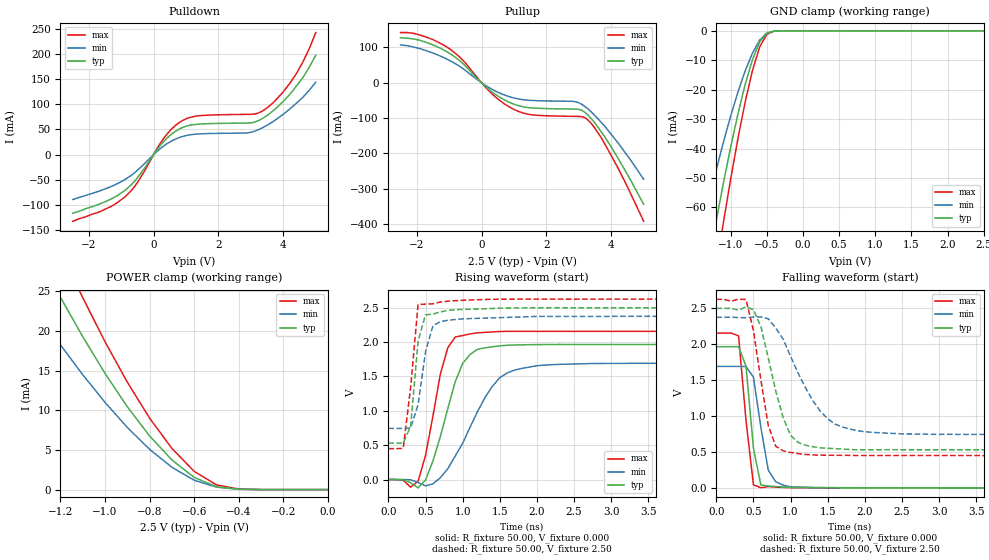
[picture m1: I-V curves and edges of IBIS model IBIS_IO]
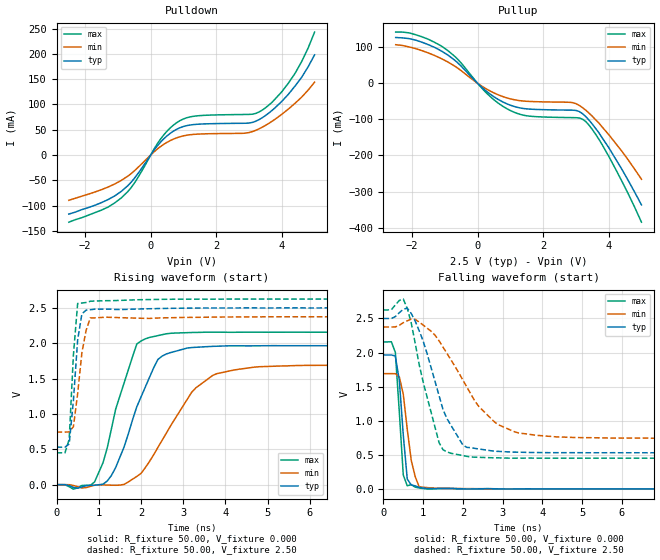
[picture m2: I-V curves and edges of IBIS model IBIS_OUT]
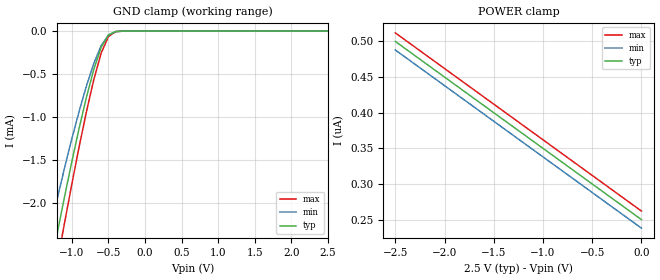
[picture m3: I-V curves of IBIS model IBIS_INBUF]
| IBIS file .ibs created by s2ibis2 version 1.1
| North Carolina State University Electronics Research Laboratory  1995
[IBIS ver]   2.1
[File name]   75602_pf.ibs
[File Rev]   1.3
[Date]   Thursday, June 28, 2001
[Source]   Integrated Device Technology, Inc.
[Notes]   1. Temperatures: typ=25C, min=100C, max=0C 2. Cemos11.5_2.5v
   process. 3. Ramp rates based on 50 ohm load.
[Copyright]   Copyright 2000, Integrated Device Technology, Inc. Integrated
   Device Technology, Inc. ("IDT") hereby grants the user of this
   IBIS model a non-exclusive, nontransferable license to use
   this IBIS model under the following terms. The user is granted
   this license only to use the IBIS model and is not granted
   rights to sell, copy (except as needed to run the IBIS model),
   rent, lease or sub-license the IBIS model in whole or in part,
   or in modified form to anyone. The User may modify the IBIS
   model to suit its specific applications, but rights to
   derivative works and such modifications shall belong to IDT.
   This IBIS model is provided on an AS IS" basis and IDT makes
   absolutely no warranty with respect to the information
   contained herein. IDT DISCLAIMS AND CUSTOMER WAIVES ALL
   WARRANTIES, EXPRESS AND IMPLIED, INCLUDING WARRANTIES OF
   MERCHANTABILITY AND FITNESS FOR A PARTICULAR PURPOSE. THE
   ENTIRE RISK AS TO QUALITY AND PERFORMANCE IS WITH THE USER
   ACCORDINGLY, IN NO EVENT SHALL IDT BE LIABLE FOR ANY DIRECT OR
   INDIRECT DAMAGES, WHETHER IN CONTRACT OR TORT, INCLUDING ANY
   LOST PROFITS OR OTHER INCIDENTAL, CONSEQUENTIAL, EXEMPLARY, OR
   PUNITIVE DAMAGES ARISING OUT OF THE USE OR APPLICATION OF THE
   IBIS model. Further, IDT reserves the right to make changes
   without notice to any product herein to improve reliability,
   function, or design. IDT does not convey any license under
   patent rights or any other intellectual property rights,
   including those of third parties. IDT is not obligated to
   provide maintenance or support for the licensed IBIS model.
|   Component IDT71T75602z_PIPELINE_ZBT_SRAM
[Component]   IDT71T75602z
[Manufacturer]   Integrated Device Technology
|   IBIS model for (PF) 100-TQFP package
[Package]
| variable   typ   min   max
R_pkg   10.00m   9.00m   11.00m
L_pkg   5.50nH   5.00nH   5.60nH
C_pkg   0.40pF   0.30pF   0.47pF
[Pin]  signal_name   model_name   R_pin   L_pin   C_pin
1   I/OP3   IBIS_IO
2   I/O16   IBIS_IO
3   I/O17   IBIS_IO
4   VDDQ   POWER
5   VSS   GND
6   I/O18   IBIS_IO
7   I/O19   IBIS_IO
8   I/O20   IBIS_IO
9   I/O21   IBIS_IO
10   VSS   GND
11   VDDQ   POWER
12   I/O22   IBIS_IO
13   I/O23   IBIS_IO
14   VDD   POWER
15   VDD   POWER
16   VDD   POWER
17   VSS   GND
18   I/O24   IBIS_IO
19   I/O25   IBIS_IO
20   VDDQ   POWER
21   VSS   GND
22   I/O26   IBIS_IO
23   I/O27   IBIS_IO
24   I/O28   IBIS_IO
25   I/O29   IBIS_IO
26   VSS   GND
27   VDDQ   POWER
28   I/O30   IBIS_IO
29   I/O31   IBIS_IO
30   I/OP4   IBIS_IO
31   LBO/   IBIS_INBUF
32   A5   IBIS_INBUF
33   A4   IBIS_INBUF
34   A3   IBIS_INBUF
35   A2   IBIS_INBUF
36   A1   IBIS_INBUF
37   A0   IBIS_INBUF
38   TMS   IBIS_INBUF
39   TDI   IBIS_INBUF
40   VSS   GND
41   VDD   POWER
42   TDO   IBIS_OUT
43   TCK   IBIS_INBUF
44   A10   IBIS_INBUF
45   A11   IBIS_INBUF
46   A12   IBIS_INBUF
47   A13   IBIS_INBUF
48   A14   IBIS_INBUF
49   A15   IBIS_INBUF
50   A16   IBIS_INBUF
51   I/OP1   IBIS_IO
52   I/O0   IBIS_IO
53   I/O1   IBIS_IO
54   VDDQ   POWER
55   VSS   GND
56   I/O2   IBIS_IO
57   I/O3   IBIS_IO
58   I/O4   IBIS_IO
59   I/O5   IBIS_IO
60   VSS   GND
61   VDDQ   POWER
62   I/O6   IBIS_IO
63   I/O7   IBIS_IO
64   ZZ   IBIS_INBUF
65   VDD   POWER
66   VDD   POWER
67   VSS   GND
68   I/O8   IBIS_IO
69   I/O9   IBIS_IO
70   VDDQ   POWER
71   VSS   GND
72   I/O10   IBIS_IO
73   I/O11   IBIS_IO
74   I/O12   IBIS_IO
75   I/O13   IBIS_IO
76   VSS   GND
77   VDDQ   POWER
78   I/O14   IBIS_IO
79   I/O15   IBIS_IO
80   I/OP2   IBIS_IO
81   A9   IBIS_INBUF
82   A8   IBIS_INBUF
83   A17   IBIS_INBUF
84   A18   IBIS_INBUF
85   ADV/LD/   IBIS_INBUF
86   OE/   IBIS_INBUF
87   CEN/   IBIS_INBUF
88   R/W/   IBIS_INBUF
89   CLK   IBIS_INBUF
90   VSS   GND
91   VDD   POWER
92   CE2/   IBIS_INBUF
93   BW1/   IBIS_INBUF
94   BW2/   IBIS_INBUF
95   BW3/   IBIS_INBUF
96   BW4/   IBIS_INBUF
97   CE2   IBIS_INBUF
98   CE1/   IBIS_INBUF
99   A7   IBIS_INBUF
100   A6   IBIS_INBUF
| Models and submodels in the file (3): IBIS_IO (I/O), IBIS_OUT (Output), IBIS_INBUF (Input)
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| in   in   dummy_model
| oel  oel   dummy_model
| int  int   dummy_model
| oelt oelt   dummy_model
|   Model IBIS_IO
[Model]   IBIS_IO
Model_type   I/O
Polarity   Non-Inverting
Enable   Active-Low
Vinl =  0.700V
Vinh =  1.700V
Vmeas =  1.250V
Cref =  0.000F
Rref = 50.000
Vref =  1.250V
C_comp   3.00pF   2.00pF   4.00pF
[Temperature Range]   25.00   100.00   0.000
[Voltage Range]   2.50V   2.37V   2.62V
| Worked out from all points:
|   slope of the pulldown table from 0 to 0.375 V, typ, clamps not added: 12.4 ohm
|   slope of the pullup table from 0 to 0.375 V, typ, clamps not added: 12.8 ohm
|   GND clamp passes 1 mA (typ) near -0.51 V on its own axis
|   POWER clamp passes 1 mA (typ) near -0.55 V on its own axis
|   rising waveform, R_fixture 50.00, V_fixture 0.000: 20-80 % time 321ps typ, 500ps min, 235ps max; typ from 0 V to 1.97 V
|   rising waveform, R_fixture 50.00, V_fixture 2.50: 20-80 % time 112ps typ, 156ps min, 122ps max; typ from 0.53 V to 2.5 V
|   falling waveform, R_fixture 50.00, V_fixture 0.000: 20-80 % time 121ps typ, 158ps min, 123ps max; typ from 1.97 V to 0 V
|   falling waveform, R_fixture 50.00, V_fixture 2.50: 20-80 % time 289ps typ, 489ps min, 197ps max; typ from 2.5 V to 0.53 V
[Pulldown]
| voltage   I(typ)   I(min)   I(max)
-2.5V     -117mA     -89.7mA    -133mA
-1.7V     -99.4mA    -73.2mA    -115mA
-900mV    -72.13mA   -50.4mA    -85.16mA
-500mV    -46.26mA   -31.43mA   -55.78mA
300mV     25.33mA    16.62mA    31.45mA
900mV     54.03mA    36.14mA    68.11mA
1.5V      61mA       41.41mA    77.8mA
3V        63.11mA    44.29mA    80.16mA
3.5V      77.88mA    58.43mA    93.16mA
4V        106mA      80.39mA    125mA
4.4V      136mA      102mA      161mA
5V        198mA      144mA      243mA
[Pullup]
| voltage   I(typ)   I(min)   I(max)
-2.5V     127mA      107mA      142mA
-1.9V     120mA      96.48mA    135mA
-1.1V     89.31mA    68.24mA    103mA
-600mV    56.27mA    41.71mA    66.02mA
300mV     -24.21mA   -17.31mA   -29.47mA
1V        -60.72mA   -43.11mA   -75.48mA
1.6V      -71.56mA   -50.32mA   -91.16mA
2.9V      -74.5mA    -53.66mA   -95.14mA
3.2V      -84.55mA   -67.99mA   -99.54mA
3.5V      -114mA     -92.99mA   -129mA
3.8V      -153mA     -123mA     -173mA
5V        -344mA     -273mA     -392mA
[GND_clamp]
| voltage   I(typ)   I(min)   I(max)
-2.5V     -256mA     -196mA     -298mA
-1.4V     -91.8mA    -67.57mA   -112mA
-1.3V     -77.92mA   -57.18mA   -96.09mA
-1.2V     -64.46mA   -47.2mA    -80.22mA
-1.1V     -51.57mA   -37.73mA   -64.88mA
-900mV    -28.17mA   -20.77mA   -36.54mA
-800mV    -18.18mA   -13.58mA   -24.15mA
-700mV    -9.823mA   -7.577mA   -13.54mA
-600mV    -3.759mA   -3.157mA   -5.506mA
-500mV    -740uA     -782uA     -1.15mA
-300mV    -2.842uA   -8.572uA   -3.594uA
2.5V      250nA      281nA      250nA
[POWER_clamp]
| voltage   I(typ)   I(min)   I(max)
-2.5V     100mA      78.58mA    117mA
-1.4V     34.98mA    26.45mA    42.72mA
-1.3V     29.51mA    22.26mA    36.31mA
-1.2V     24.26mA    18.26mA    30.12mA
-1.1V     19.29mA    14.49mA    24.21mA
-900mV    10.45mA    7.838mA    13.55mA
-800mV    6.77mA     5.078mA    9.014mA
-700mV    3.737mA    2.813mA    5.196mA
-600mV    1.535mA    1.182mA    2.3mA
-500mV    362uA      310uA      599uA
-400mV    41.18uA    46.02uA    69.44uA
0V        250nA      239nA      262nA
[Ramp]
| variable   typ   min   max
dV/dt_r   1.18/0.30n   1.02/0.49n   1.30/0.22n
dV/dt_f   1.18/0.28n   0.98/0.50n   1.31/0.21n
R_load = 50.00
[Rising Waveform]
R_fixture = 50.00
V_fixture = 0.000
V_fixture_min = 0.000
V_fixture_max = 0.000
C_fixture = 0.000F
R_dut = 68.00m
L_dut = 2.31nH
C_dut = 0.65pF
| time   V(typ)   V(min)   V(max)
0s        0V         0V         0V
300ps     -45.68mV   -3.202mV   -111mV
400ps     -121mV     -43.62mV   -25.43mV
500ps     -8.692mV   -91.97mV   351mV
700ps     627mV      26.44mV    1.537V
800ps     1.032V     157mV      1.917V
1.1ns     1.819V     763mV      2.119V
1.5ns     1.945V     1.482V     2.154V
2ns       1.963V     1.656V     2.156V
9.9ns     1.965V     1.691V     2.156V
[Rising Waveform]
R_fixture = 50.00
V_fixture = 2.50
V_fixture_min = 2.37
V_fixture_max = 2.62
C_fixture = 0.000F
R_dut = 68.00m
L_dut = 2.31nH
C_dut = 0.65pF
| time   V(typ)   V(min)   V(max)
0s        530mV      744mV      450mV
200ps     530mV      744mV      453mV
300ps     777mV      750mV      1.343V
400ps     2.017V     1.09V      2.547V
500ps     2.397V     1.859V     2.552V
600ps     2.407V     2.239V     2.557V
700ps     2.44V      2.298V     2.583V
800ps     2.46V      2.318V     2.595V
2ns       2.499V     2.373V     2.625V
9.9ns     2.5V       2.375V     2.625V
[Falling Waveform]
R_fixture = 50.00
V_fixture = 0.000
V_fixture_min = 0.000
V_fixture_max = 0.000
C_fixture = 0.000F
R_dut = 68.00m
L_dut = 2.31nH
C_dut = 0.65pF
| time   V(typ)   V(min)   V(max)
0s        1.965V     1.691V     2.156V
200ps     1.965V     1.691V     2.156V
300ps     1.966V     1.691V     2.116V
400ps     1.694V     1.689V     939mV
500ps     556mV      1.541V     41.85mV
600ps     40.07mV    844mV      1.621mV
700ps     25.66mV    246mV      17.7mV
800ps     17.72mV    84.79mV    10.16mV
1ns       6.48mV     15.89mV    3.136mV
9.9ns     -347nV     1.011uV    -1.87uV
[Falling Waveform]
R_fixture = 50.00
V_fixture = 2.50
V_fixture_min = 2.37
V_fixture_max = 2.62
C_fixture = 0.000F
R_dut = 68.00m
L_dut = 2.31nH
C_dut = 0.65pF
| time   V(typ)   V(min)   V(max)
0s        2.5V       2.375V     2.625V
400ps     2.52V      2.368V     2.623V
500ps     2.481V     2.379V     2.19V
600ps     2.246V     2.381V     1.503V
700ps     1.808V     2.354V     867mV
800ps     1.349V     2.225V     580mV
1ns       730mV      1.83V      492mV
1.5ns     551mV      961mV      454mV
2ns       530mV      781mV      450mV
9.9ns     530mV      744mV      450mV
|   Model IBIS_OUT
[Model]   IBIS_OUT
Model_type   Output
Polarity   Non-Inverting
Enable   Active-Low
Vmeas =  1.250V
Cref =  0.000F
Rref = 50.000
Vref =  1.250V
C_comp   3.00pF   2.00pF   4.00pF
[Temperature Range]   25.00   100.00   0.000
[Voltage Range]   2.50V   2.37V   2.62V
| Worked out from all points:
|   slope of the pulldown table from 0 to 0.375 V, typ, clamps not added: 12.4 ohm
|   slope of the pullup table from 0 to 0.375 V, typ, clamps not added: 12.8 ohm
|   rising waveform, R_fixture 50.00, V_fixture 0.000: 20-80 % time 737ps typ, 1.06ns min, 595ps max; typ from 0 V to 1.97 V
|   rising waveform, R_fixture 50.00, V_fixture 2.50: 20-80 % time 160ps typ, 204ps min, 128ps max; typ from 0.53 V to 2.5 V
|   falling waveform, R_fixture 50.00, V_fixture 0.000: 20-80 % time 159ps typ, 227ps min, 143ps max; typ from 1.97 V to 0 V
|   falling waveform, R_fixture 50.00, V_fixture 2.50: 20-80 % time 675ps typ, 1.11ns min, 525ps max; typ from 2.5 V to 0.53 V
[Pulldown]
| voltage   I(typ)   I(min)   I(max)
-2.5V     -117mA     -89.7mA    -133mA
-1.5V     -94.2mA    -68.59mA   -109mA
-900mV    -72.12mA   -50.41mA   -85.11mA
-500mV    -46.26mA   -31.43mA   -55.77mA
300mV     25.33mA    16.62mA    31.45mA
900mV     54.03mA    36.14mA    68.11mA
1.5V      61mA       41.41mA    77.8mA
3V        63.11mA    44.29mA    80.16mA
3.5V      77.88mA    58.43mA    93.16mA
4V        106mA      80.39mA    125mA
4.4V      136mA      102mA      161mA
5V        198mA      144mA      243mA
[Pullup]
| voltage   I(typ)   I(min)   I(max)
-2.5V     127mA      107mA      142mA
-1.9V     120mA      96.48mA    135mA
-1.1V     89.31mA    68.24mA    103mA
-600mV    56.27mA    41.71mA    66.02mA
300mV     -24.21mA   -17.31mA   -29.47mA
1V        -60.72mA   -43.11mA   -75.48mA
1.6V      -71.56mA   -50.32mA   -91.16mA
2.9V      -74.49mA   -53.6mA    -95.14mA
3.3V      -92.23mA   -74.49mA   -106mA
3.6V      -125mA     -101mA     -141mA
4V        -178mA     -142mA     -202mA
5V        -337mA     -266mA     -385mA
[Ramp]
| variable   typ   min   max
dV/dt_r   1.18/0.74n   1.02/1.05n   1.30/0.61n
dV/dt_f   1.18/0.66n   0.98/1.11n   1.31/0.53n
R_load = 50.00
[Rising Waveform]
R_fixture = 50.00
V_fixture = 0.000
V_fixture_min = 0.000
V_fixture_max = 0.000
C_fixture = 0.000F
R_dut = 68.00m
L_dut = 2.31nH
C_dut = 0.65pF
| time   V(typ)   V(min)   V(max)
0s        0V         0V         0V
900ps     -8.624mV   -8.352mV   38.26mV
1.1ns     6.189mV    -4.095mV   309mV
1.4ns     242mV      -8.698mV   1.068V
1.9ns     1.101V     116mV      1.988V
2.1ns     1.378V     239mV      2.062V
2.5ns     1.818V     628mV      2.121V
3.2ns     1.939V     1.307V     2.152V
3.8ns     1.958V     1.571V     2.157V
9.9ns     1.965V     1.691V     2.156V
[Rising Waveform]
R_fixture = 50.00
V_fixture = 2.50
V_fixture_min = 2.37
V_fixture_max = 2.62
C_fixture = 0.000F
R_dut = 68.00m
L_dut = 2.31nH
C_dut = 0.65pF
| time   V(typ)   V(min)   V(max)
0s        530mV      744mV      450mV
200ps     530mV      744mV      450mV
300ps     576mV      745mV      642mV
400ps     1.192V     821mV      1.837V
500ps     2.047V     1.285V     2.562V
600ps     2.415V     1.865V     2.569V
700ps     2.468V     2.182V     2.577V
800ps     2.474V     2.359V     2.594V
2.9ns     2.495V     2.364V     2.624V
9.9ns     2.5V       2.375V     2.625V
[Falling Waveform]
R_fixture = 50.00
V_fixture = 0.000
V_fixture_min = 0.000
V_fixture_max = 0.000
C_fixture = 0.000F
R_dut = 68.00m
L_dut = 2.31nH
C_dut = 0.65pF
| time   V(typ)   V(min)   V(max)
0s        1.965V     1.691V     2.156V
200ps     1.965V     1.691V     2.159V
300ps     1.948V     1.69V      2.004V
400ps     1.593V     1.644V     1.13V
500ps     790mV      1.388V     203mV
600ps     144mV      875mV      45.08mV
700ps     58.18mV    420mV      62.05mV
800ps     44.52mV    179mV      25.37mV
900ps     21.3mV     29.52mV    12.94mV
9.9ns     26.72uV    503nV      67.94uV
[Falling Waveform]
R_fixture = 50.00
V_fixture = 2.50
V_fixture_min = 2.37
V_fixture_max = 2.62
C_fixture = 0.000F
R_dut = 68.00m
L_dut = 2.31nH
C_dut = 0.65pF
| time   V(typ)   V(min)   V(max)
0s        2.5V       2.375V     2.625V
500ps     2.634V     2.438V     2.785V
800ps     2.462V     2.487V     2.137V
1ns       2.169V     2.403V     1.568V
1.4ns     1.368V     2.173V     678mV
1.6ns     1.029V     1.986V     542mV
2.1ns     609mV      1.493V     477mV
2.8ns     552mV      979mV      456mV
3.4ns     538mV      821mV      451mV
9.9ns     530mV      743mV      450mV
|   Model IBIS_INBUF
[Model]   IBIS_INBUF
Model_type   Input
Vinl =  0.700V
Vinh =  1.700V
Vmeas =  1.250V
C_comp   1.00pF   0.80pF   1.20pF
[Temperature Range]   25.00   100.00   0.000
[Voltage Range]   2.50V   2.37V   2.62V
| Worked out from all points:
|   GND clamp passes 1 mA (typ) near -0.86 V on its own axis
[GND_clamp]
| voltage   I(typ)   I(min)   I(max)
-2.5V     -8.52mA    -7.269mA   -9.344mA
-1.3V     -2.8mA     -2.326mA   -3.189mA
-1.2V     -2.361mA   -1.956mA   -2.709mA
-1.1V     -1.934mA   -1.599mA   -2.24mA
-900mV    -1.133mA   -935uA     -1.349mA
-800mV    -770uA     -639uA     -939uA
-700mV    -448uA     -378uA     -567uA
-600mV    -192uA     -171uA     -259uA
-500mV    -43.53uA   -47.01uA   -64.09uA
-400mV    -4.09uA    -6.592uA   -5.956uA
-300mV    -207nA     -579nA     -248nA
2.5V      250nA      250nA      250nA
[POWER_clamp]
| voltage   I(typ)   I(min)   I(max)
-2.5V     500nA      488nA      512nA
-2.3V     480nA      468nA      492nA
-2.1V     460nA      448nA      472nA
0V        250nA      238nA      262nA
